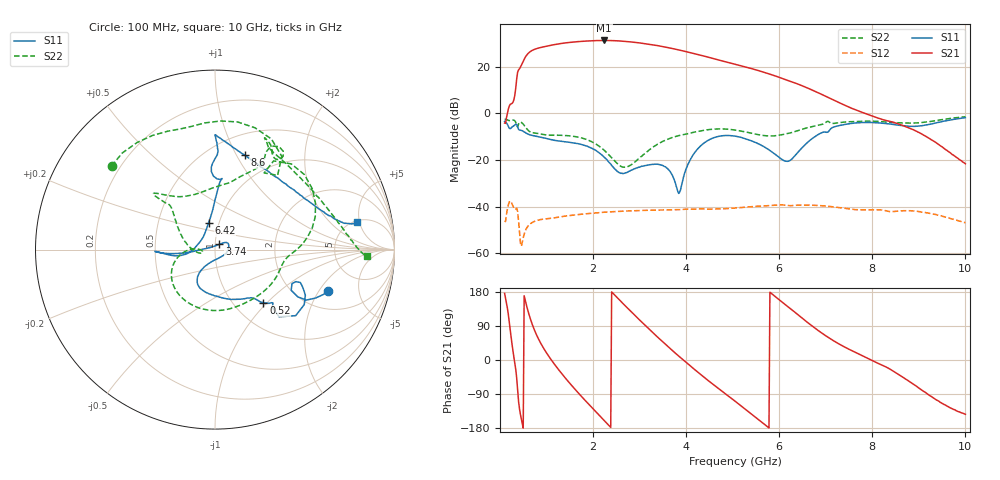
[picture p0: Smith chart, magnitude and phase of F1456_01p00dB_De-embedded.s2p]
! Integrated Device Technology
! Corporate Headquarters
! 6024 Silver Creek Valley Road
! San Jose, CA 95138  USA
! Phone:  1-408-284-8200
! Toll Free:  1-800-223-1366
! Webpage:  http://www.idt.com/
! Timing and RF Division
! 515 Groton Road, Suite 102
! Westford, MA 01886-6024
! Device:  F1456
! Description: 6-bit 0.5 dB Transmit Variable Gain Amplifier
! Frequency:  2100.0 -  2950.00 MHz
! Package:  6x6 mm Thin QFN Plastic Package: 28 pin
! State:  2
! Atten State:  1.0 dB
! Voltage:  +5.00 Volts
! Current:  213.500 mA
! Data:  The device was measured on a the F1455 evaluation board which has
!  individual transmission lines to the RF pins.  Data was collected
!  using a calibrated network analyzer.  The evaluation board was
!  de-embedded using a TRL calibration technique.
!  The reference plane is the edge of the package pin.
!  Pin  1 = CSb
!  Pin  2 = DATA
!  Pin  3 = CLK
!  Pin  4 = RSET
!  Pin  5 = GND
!  Pin  6 = RFIN  = Port 1
!  Pin  7 = GND
!  Pin  8 = NC
!  Pin  9 = NC
!  Pin 10 = NC
!  Pin 11 = NC
!  Pin 12 = NC
!  Pin 13 = NC
!  Pin 14 = /STBY
!  Pin 15 = GND
!  Pin 16 = RFOUT  = Port 2
!  Pin 17 = GND
!  Pin 18 = NC
!  Pin 19 = NC
!  Pin 20 = NC
!  Pin 21 = GND
!  Pin 22 = NC
!  Pin 23 = GND
!  Pin 24 = NC
!  Pin 25 = NC
!  Pin 26 = NC
!  Pin 27 = GND
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# GHz S dB R 50
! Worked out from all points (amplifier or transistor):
!   496 points, 100 MHz to 10 GHz, reference 50 ohm
!   highest |S21| = 31.3 dB at 2.24 GHz (marker M1)
!   |S21| within 3 dB of that: 879.5 MHz to 3.591 GHz (2.711 GHz wide, 121 % of centre)
!   unconditionally stable (mu >= 1): start of sweep to end of sweep
!   at 1.74 GHz: K = 1.99, MAG = 31.4 dB, |S12| = -43.3 dB
!   at 5.06 GHz: K = 3.64, MAG = 22.3 dB, |S12| = -40.6 dB
!   at 10 GHz: K = 134.45, MAG = -11.6 dB, |S12| = -47.0 dB
!   S11 on the Smith chart (normalised r, x): 100 MHz: 2.88, -2.42; 520 MHz: 1.35, -0.95; 3.74 GHz: 1.05, +0.06; 6.42 GHz: 0.89, +0.27; 8.6 GHz: 0.71, +1.08; 10 GHz: 5.25, +4.61
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0.1  -3.47 -20.2  -4.15 175.8  -46.24 41.2  -2.61 141.1
0.34  -4.67 -31.7  10.97 -25.3  -41.04 -141.0  -3.89 54.4
0.42  -7.15 -42.6  19.19 -129.1  -51.15 140.0  -3.89 48.3
0.52  -7.95 -47.6  23.27 169.6  -51.87 -162.4  -5.11 12.5
0.64  -9.20 -51.4  26.37 113.8  -47.63 161.8  -7.83 -5.8
0.76  -9.76 -56.2  27.63 73.5  -46.22 129.9  -8.47 -19.8
0.94  -10.52 -68.8  28.60 30.6  -45.39 95.7  -9.10 -47.1
1.12  -11.36 -82.2  29.36 -2.7  -45.00 73.9  -9.38 -72.4
1.46  -12.32 -103.1  30.40 -55.7  -43.96 45.5  -9.58 -115.5
1.76  -13.41 -117.1  30.94 -97.3  -43.29 25.7  -10.57 -143.9
2.24  -18.80 -121.9  31.32 -159.8  -42.45 -1.4  -15.85 -177.3
2.52  -24.96 -89.8  31.17 164.5  -42.12 -16.3  -21.54 -179.9
2.86  -24.06 -21.4  30.59 122.4  -41.83 -33.2  -21.45 -166.8
3.4  -21.86 25.8  29.04 58.9  -41.51 -58.9  -13.11 152.9
3.74  -28.33 49.7  27.70 21.1  -41.40 -73.8  -10.12 138.4
4.36  -13.09 -174.2  24.76 -43.1  -41.06 -101.8  -7.32 137.9
5.06  -9.79 -177.9  21.06 -109.5  -40.64 -129.9  -7.18 134.8
6.42  -16.32 103.2  12.44 117.6  -39.38 152.5  -7.24 70.4
6.7  -10.94 89.6  10.10 90.4  -39.41 133.4  -5.71 62.4
8.36  -4.51 83.0  -3.34 -22.6  -42.14 60.0  -3.83 62.5
8.6  -5.16 72.6  -4.81 -41.1  -41.89 54.3  -4.07 55.8
10  -1.86 10.9  -21.64 -143.3  -46.95 -21.2  -1.46 -2.5
